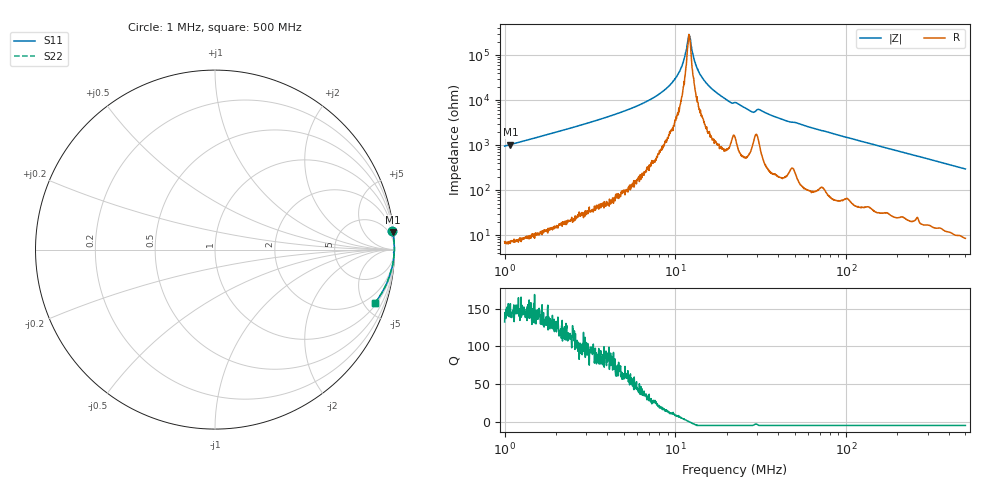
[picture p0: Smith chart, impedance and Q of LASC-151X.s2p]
!s-Parameter Generated by FASTRON Sdn. Bhd.
!FASTRON P/N : LASC-151X
!Keysight Technologies,E4991B,MY54100416,A.01.15
!Date: Tue Mar 17 15:06:44 2026
!Version  : Rev00 Tue Mar 17 15:06:44 2026
!Data & Calibration Information:
!PortZ  Port1:50+j0  Port2:50+j0
!When reading, reference impedance value at option line is always used.
! Remarks : This data is being provided solely for informational purposes.
!Freq	S11	S21	S12	S22
# Hz S dB R 50
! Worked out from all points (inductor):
!   1601 points, 1 MHz to 500 MHz, reference 50 ohm
!   read as one part in series: L = 150 uH near 1.032 MHz
!   highest Q = 150 at 1.081 MHz (marker M1), where L = 151 uH
!   self-resonance near 12.01 MHz
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1000000  -0.05 6.0  -19.60 -83.6  -19.60 -83.6  -0.05 6.0
1080780  -0.05 5.6  -20.27 -84.1  -20.27 -84.1  -0.05 5.6
2820919  -0.01 2.0  -28.98 -87.4  -28.98 -87.4  -0.01 2.0
5396294  -0.00 0.9  -36.01 -87.9  -36.01 -87.9  -0.00 0.9
7957584  -0.00 0.4  -42.46 -86.8  -42.46 -86.8  -0.00 0.4
9331304  -0.00 0.3  -46.82 -84.9  -46.82 -84.9  -0.00 0.3
1.036305e7  -0.00 0.2  -51.43 -82.1  -51.43 -82.1  -0.00 0.2
1.10275e7  -0.00 0.1  -56.05 -76.5  -56.05 -76.5  -0.00 0.1
1.178023e7  -0.00 0.0  -65.57 -43.0  -65.57 -43.0  -0.00 0.0
1.205799e7  -0.00 -0.0  -68.06 4.9  -68.06 4.9  -0.00 -0.0
1.229445e7  -0.00 -0.0  -66.22 44.0  -66.22 44.0  -0.00 -0.0
1.288105e7  -0.00 -0.1  -58.33 73.4  -58.33 73.4  -0.00 -0.1
1.33393e7  -0.00 -0.1  -54.59 79.1  -54.59 79.1  -0.00 -0.1
1.475677e7  -0.00 -0.2  -48.73 83.0  -48.73 83.0  -0.00 -0.2
1.820043e7  -0.01 -0.4  -42.24 85.5  -42.24 85.5  -0.01 -0.4
2.093189e7  -0.01 -0.6  -39.10 83.1  -39.10 83.1  -0.01 -0.6
2.236068e7  -0.02 -0.6  -38.93 79.5  -38.93 79.5  -0.02 -0.6
2.811962e7  -0.03 -1.0  -34.78 79.6  -34.78 79.6  -0.03 -1.0
3.110769e7  -0.02 -0.9  -35.77 79.7  -35.77 79.7  -0.02 -0.9
6.307767e7  -0.02 -2.4  -27.66 85.4  -27.66 85.4  -0.02 -2.4
1.77937e8  -0.10 -6.8  -18.55 81.2  -18.55 81.2  -0.10 -6.8
5e8  -0.55 -18.6  -9.94 69.8  -9.94 69.8  -0.55 -18.6
